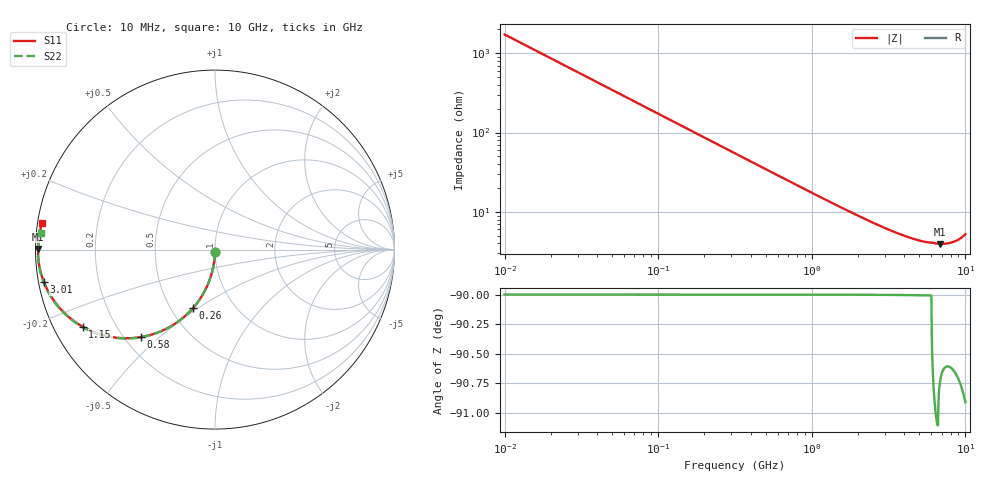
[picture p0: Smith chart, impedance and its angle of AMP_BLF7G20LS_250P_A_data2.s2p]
! Created Thu Oct 28 10:30:21 2010
# ghz S ma R 50
! 2 Port Network Data from SP1.SP block
! freq  magS11  angS11  magS21  angS21  magS12  angS12  magS22  angS22
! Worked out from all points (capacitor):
!   1000 points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, 10 MHz to 10 GHz, reference 50 ohm
!   read as one part in shunt: C = 9.21 pF near 60 MHz
!   lowest |Z| = 3.95 ohm at 6.85 GHz (marker M1)
!   S11 on the Smith chart (normalised r, x): 10 MHz: 1.00, -0.03; 260 MHz: 0.64, -0.48; 580 MHz: 0.26, -0.44; 1.15 GHz: 0.09, -0.27; 3.01 GHz: 0.02, -0.09; 10 GHz: 0.01, +0.08
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0.01  0.01439 -90.8  0.9999 -0.8  0.9999 -0.8  0.01439 -90.8
0.04  0.05748 -93.3  0.9983 -3.3  0.9983 -3.3  0.05748 -93.3
0.07  0.1002 -95.8  0.995 -5.8  0.995 -5.8  0.1002 -95.8
0.09  0.1285 -97.5  0.9917 -7.5  0.9917 -7.5  0.1285 -97.5
0.11  0.1564 -99.1  0.9877 -9.1  0.9877 -9.1  0.1564 -99.1
0.14  0.1975 -101.5  0.9803 -11.5  0.9803 -11.5  0.1975 -101.5
0.17  0.2376 -103.9  0.9714 -13.9  0.9714 -13.9  0.2376 -103.9
0.26  0.3503 -110.8  0.9366 -20.7  0.9366 -20.7  0.3503 -110.7
0.4  0.4983 -120.3  0.867 -30.3  0.867 -30.3  0.4983 -120.2
0.58  0.6396 -130.3  0.7687 -40.3  0.7687 -40.3  0.6396 -130.2
0.85  0.7721 -141.4  0.6355 -51.3  0.6355 -51.3  0.7721 -141.2
1.15  0.853 -149.7  0.5218 -59.6  0.5218 -59.6  0.853 -149.5
1.39  0.8912 -154.5  0.4536 -64.3  0.4536 -64.3  0.8912 -154.2
1.68  0.9205 -158.7  0.3907 -68.6  0.3907 -68.6  0.9205 -158.4
2.24  0.9511 -164.4  0.3089 -74.1  0.3089 -74.1  0.9511 -163.9
3.01  0.97 -169.2  0.2432 -78.9  0.2432 -78.9  0.97 -168.5
3.34  0.9745 -170.7  0.2244 -80.3  0.2244 -80.3  0.9745 -170.0
5.01  0.985 -176.1  0.1726 -85.5  0.1726 -85.5  0.985 -174.9
6.67  0.9846 -179.8  0.1565 -89.9  0.1565 -89.9  0.9855 -178.1
6.85  0.9852 179.8  0.1565 -90.1  0.1565 -90.1  0.986 -178.5
8.34  0.9839 176.4  0.1657 -93.1  0.1657 -93.1  0.9846 178.7
10  0.9747 171.3  0.2059 -98.0  0.2059 -98.0  0.9758 174.7
